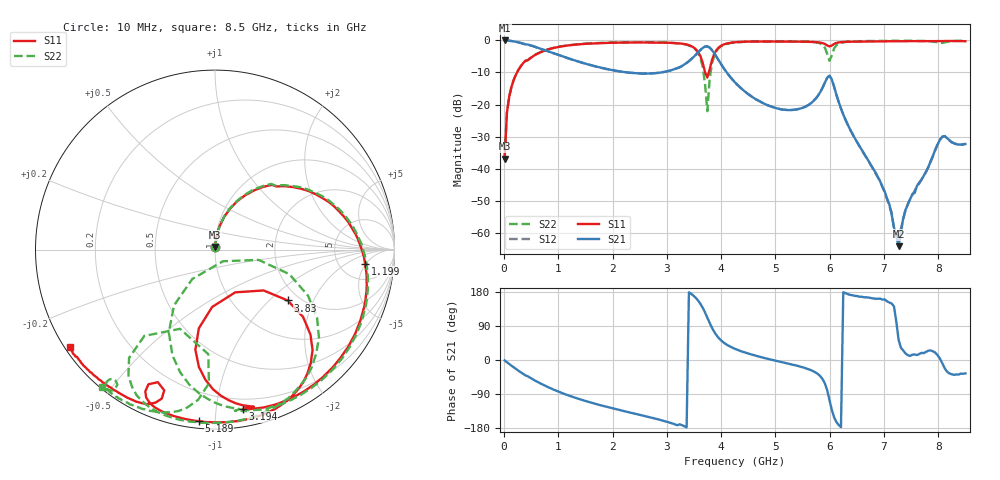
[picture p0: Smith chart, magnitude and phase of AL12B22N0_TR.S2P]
!AVX CORPORATION
!PART NUMBER AL12B22N0_TR
!DESCRIPTION: AIR CORE INDUCTOR, 22nH, 7 TURNS
!Agilent Technologies,E5071C,MY46102230,A.09.54
!Date: Mon Sep 03 15:59:33 2012
!Data & Calibration Information:
!Freq	S11:SOLT2(ON)	S21:SOLT2(ON)	S12:SOLT2(ON)	S22:SOLT2(ON)
# Hz S RI R 50
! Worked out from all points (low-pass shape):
!   201 points, 10 MHz to 8.5 GHz, reference 50 ohm
!   highest |S21| = -0.01 dB at 10 MHz (marker M1); lowest = -64.2 dB at 7.269 GHz (marker M2)
!   |S21| within 3 dB of the highest: start of sweep to 744.9 MHz; 3.617 GHz to 3.831 GHz (214.4 MHz wide, 5.76 % of centre)
!   lowest |S11| = -36.9 dB at 10 MHz (marker M3), VSWR 1.03, Z = 50 + j1.43 ohm
!   |S11| at or under -10 dB: start of sweep to 239.2 MHz; 3.706 GHz to 3.772 GHz (66.24 MHz wide, 1.77 % of centre)
!   |S22| runs from -36.7 to -0.1 dB; largest |S21 - S12| = 0.01
!   S11 on the Smith chart (normalised r, x): 10 MHz: 1.00, +0.03; 1.199 GHz: 9, -5; 3.194 GHz: 0.13, -1.18; 3.83 GHz: 1.74, -1.31; 5.189 GHz: 0.04, -0.91; 8.5 GHz: 0.01, -0.30
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1e7  0.000471 0.0143  0.9992 -0.02  0.9942 -0.029  0.000508 0.0147
5.245e7  0.00818 0.0737  0.9911 -0.1014  0.9938 -0.1024  0.00828 0.0741
9.49e7  0.0254 0.13  0.9721 -0.1799  0.9745 -0.1794  0.0256 0.1305
2.647e8  0.1688 0.3032  0.8217 -0.4413  0.8232 -0.4425  0.1656 0.3057
1.1986e9  0.8361 -0.0782  -0.0374 -0.5193  -0.038 -0.5194  0.8418 -0.0625
1.4533e9  0.8403 -0.2606  -0.1236 -0.4278  -0.1244 -0.4281  0.8489 -0.2503
2.85415e9  0.3719 -0.8507  -0.2883 -0.1214  -0.2881 -0.1212  0.3408 -0.8704
3.19375e9  0.1536 -0.8876  -0.3684 -0.0509  -0.3685 -0.0508  0.1108 -0.898
3.61825e9  -0.1094 -0.5577  -0.6027 0.3752  -0.6027 0.3756  -0.2571 -0.4614
3.7456e9  0.1128 -0.2381  -0.2974 0.7507  -0.297 0.7511  0.0448 -0.0648
3.8305e9  0.4051 -0.2834  0.0599 0.7059  0.0602 0.7061  0.4138 -0.1365
4.255e9  0.3837 -0.8543  0.1931 0.1089  0.193 0.1086  0.3745 -0.8501
5.1889e9  -0.0904 -0.9557  0.0816 -0.0116  0.0817 -0.0117  -0.1418 -0.9585
5.6983e9  -0.3111 -0.8931  0.098 -0.0562  0.0983 -0.0562  -0.3859 -0.8616
5.91055e9  -0.3885 -0.7905  0.1043 -0.1929  0.1041 -0.1927  -0.4787 -0.6034
5.99545e9  -0.3185 -0.7386  -0.0719 -0.272  -0.0718 -0.2721  -0.1951 -0.4414
6.2077e9  -0.3829 -0.8603  -0.0864 -0.00447  -0.0863 -0.00462  -0.2011 -0.8987
7.09915e9  -0.644 -0.7253  -0.00244 0.00131  -0.00233 0.00115  -0.5206 -0.8384
7.26895e9  -0.6738 -0.7006  0.000365 0.000497  0.000486 0.000848  -0.5439 -0.8214
7.3963e9  -0.6951 -0.6828  0.00217 0.000683  0.00216 0.000571  -0.5617 -0.8107
8.03305e9  -0.768 -0.5985  0.0285 0.00156  0.0282 0.00186  -0.5735 -0.7192
8.5e9  -0.8097 -0.5404  0.0197 -0.014  0.02 -0.0141  -0.6278 -0.766
